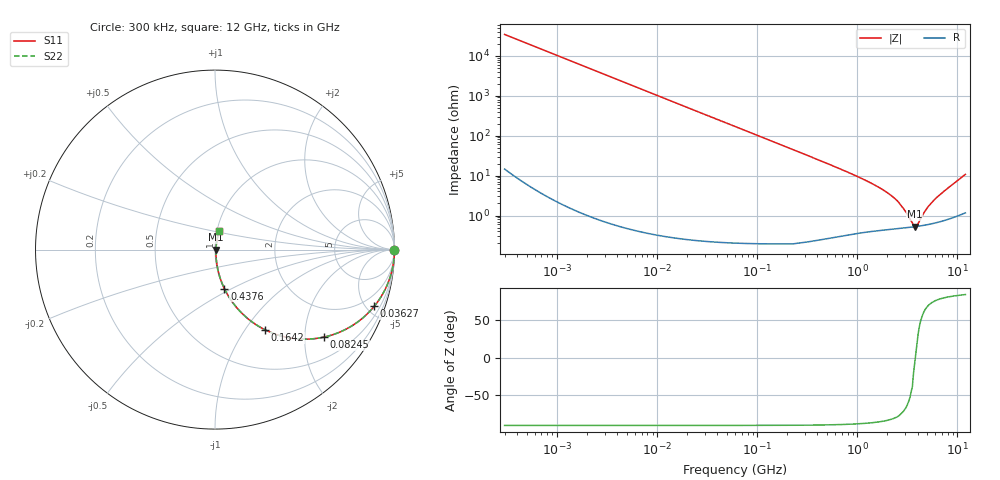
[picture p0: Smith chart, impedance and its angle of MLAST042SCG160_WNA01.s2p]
! MLAST042SCG160_WNA01  S-PARAMETER MODEL  ( General Type )
! Model Generated by TAIYO YUDEN Corporation (http://www.ty-top.com)
! Version 1.0
! TAIYO YUDEN Control No. 150820
! Copyright(c) 2015 TAIYO YUDEN CO.,LTD. All Rights Reserved.
! Product Description (link to TY-COMPAS)
! https://ds.yuden.co.jp/TYCOMPAS/or/detail?pn=MLAST042SCG160JWNA01&u=M
! Products Name : Multilayer Ceramic Capacitors
! Characteristics :
!  Capacitance : 16 pF , Rated Voltage : 25V , TCC : CG / C0G
!  Case Size : 0.4 x 0.2 / 0.016 x 0.008 [mm/inch] , Thickness : 0.2 / 0.008 [mm/inch]
!  (Conditions: Temperature = 25 degC , DC Bias Current/Voltage = 0A / 0V)
! External Node Assignments :
!  1  o---| |---o  2
! GND o---------o GND
! Frequency Range : 0.3MHz  -  12000MHz  [ 401 STEP ]
# MHz S RI R 50
! Freq[MHz].  S11 Real  S11 Imag  S21 Real  S21 Imag  S12 Real  S12 Imag  S22 Real  S22 Imag
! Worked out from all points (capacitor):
!   401 points, 300 kHz to 12 GHz, reference 50 ohm
!   read as one part in series: C = 15.6 pF near 316.3 kHz
!   lowest |Z| = 527 mohm at 3.741 GHz (marker M1)
!   series resonance near 3.789 GHz, so ESL is about 110 pH
!   S11 on the Smith chart (normalised r, x): 300 kHz: open; 36.27 MHz: 1.00, -5.63; 82.45 MHz: 1.00, -2.47; 164.2 MHz: 1.00, -1.24; 437.6 MHz: 1.00, -0.46; 12 GHz: 1.02, +0.21
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0.3  1 -0.00294  9.9e-06 0.00294  9.9e-06 0.00294  1 -0.00294
1.769972  0.9997 -0.0173  0.000304 0.0173  0.000304 0.0173  0.9997 -0.0173
10.44266  0.9896 -0.1013  0.0104 0.1013  0.0104 0.1013  0.9896 -0.1013
21.35258  0.958 -0.2004  0.042 0.2004  0.042 0.2004  0.958 -0.2004
36.27049  0.8876 -0.3154  0.1124 0.3154  0.1124 0.3154  0.8876 -0.3154
60  0.7427 -0.4365  0.2573 0.4365  0.2573 0.4365  0.7427 -0.4365
82.45425  0.6046 -0.4881  0.3954 0.4881  0.3954 0.4881  0.6046 -0.4881
116.3536  0.4344 -0.4946  0.5656 0.4946  0.5656 0.4946  0.4344 -0.4946
164.1901  0.2785 -0.4467  0.7215 0.4467  0.7215 0.4467  0.2785 -0.4467
237.9135  0.1555 -0.3601  0.8445 0.3601  0.8445 0.3601  0.1555 -0.3601
353.9943  0.0773 -0.2631  0.9227 0.2631  0.9227 0.2631  0.0773 -0.2631
437.5599  0.0524 -0.2175  0.9476 0.2175  0.9476 0.2175  0.0524 -0.2175
1166.079  0.00992 -0.0781  0.9901 0.0781  0.9901 0.0781  0.00992 -0.0781
2088.533  0.00558 -0.0337  0.9944 0.0337  0.9944 0.0337  0.00558 -0.0337
2650.866  0.00507 -0.0189  0.9949 0.0189  0.9949 0.0189  0.00507 -0.0189
3026.31  0.00501 -0.0116  0.995 0.0116  0.995 0.0116  0.00501 -0.0116
3547.679  0.00513 -0.00401  0.9949 0.00401  0.9949 0.00401  0.00513 -0.00401
3740.715  0.0052 -0.000639  0.9948 0.000639  0.9948 0.000639  0.0052 -0.000639
3944.255  0.00531 0.00189  0.9947 -0.00189  0.9947 -0.00189  0.00531 0.00189
4875.354  0.00595 0.0129  0.994 -0.0129  0.994 -0.0129  0.00595 0.0129
5868.704  0.00693 0.0235  0.9931 -0.0235  0.9931 -0.0235  0.00693 0.0235
12000  0.0224 0.103  0.9776 -0.103  0.9776 -0.103  0.0224 0.103
